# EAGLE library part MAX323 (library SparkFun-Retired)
RETIRED Dual low-voltage SPST analog switch
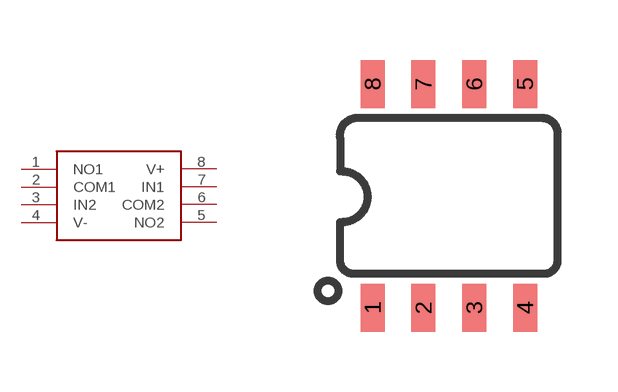
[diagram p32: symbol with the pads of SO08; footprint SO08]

Designator prefix U

## MAX323 (PROD_ID: IC-08171; VALUE: MAX323)  [SO08]
1  NO1
2  COM1
3  IN2
4  V-
5  NO2
6  COM2
7  IN1
8  V+

## Footprint SO08 (pad centres in mm)
SOIC, 0.15 inch width
smd 0.6 x 1.2: 1 -1.905,-2.8; 2 -0.635,-2.8; 3 0.635,-2.8; 4 1.905,-2.8; 5 1.905,2.8; 6 0.635,2.8; 7 -0.635,2.8; 8 -1.905,2.8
